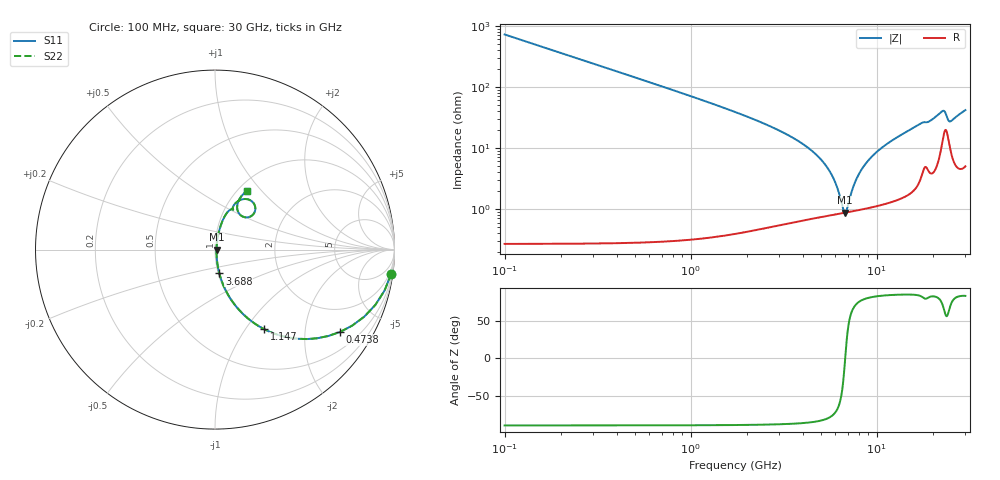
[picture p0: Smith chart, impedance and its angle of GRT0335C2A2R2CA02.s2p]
!Murata Part Number: GRT0335C2A2R2CA02
!These Parameters are Measured in Series Mode Connection
!Data Generated on Jun 19, 2026
!  o--ll--o
!Port1  Port2
!  o------o
!Operation Temp=25[degC], DC Bias Voltage=0[V]
!Freq. Start=100[MHz] Stop=30[GHz] 401[Steps]
# Hz S RI R 50
!Freq.(Hz) S11(Real) S11(Imag) S21(Real) S21(Imag) S12(Real) S12(Imag) S22(Real) S22(Imag)
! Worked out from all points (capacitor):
!   401 points, 100 MHz to 30 GHz, reference 50 ohm
!   read as one part in series: C = 2.2 pF near 249.5 MHz
!   lowest |Z| = 871 mohm at 6.753 GHz (marker M1)
!   series resonance near 6.776 GHz, so ESL is about 250 pH
!   S11 on the Smith chart (normalised r, x): 100 MHz: 1, -14; 473.8 MHz: 1.01, -3.04; 1.147 GHz: 1.01, -1.22; 3.688 GHz: 1.01, -0.27; 30 GHz: 1.10, +0.83
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1e8  0.9812 -0.1357  0.0188 0.1357  0.0188 0.1357  0.9812 -0.1357
3.2425e8  0.8317 -0.3735  0.1683 0.3735  0.1683 0.3735  0.8317 -0.3735
4.7375e8  0.6973 -0.4585  0.3027 0.4585  0.3027 0.4585  0.6973 -0.4585
7.7275e8  0.4602 -0.4968  0.5398 0.4968  0.5398 0.4968  0.4602 -0.4968
1.1465e9  0.2734 -0.443  0.7266 0.443  0.7266 0.443  0.2734 -0.443
2.0435e9  0.0961 -0.2882  0.9039 0.2882  0.9039 0.2882  0.0961 -0.2882
3.688e9  0.0241 -0.1326  0.9759 0.1326  0.9759 0.1326  0.0241 -0.1326
5.10825e9  0.0109 -0.0593  0.9891 0.0593  0.9891 0.0593  0.0109 -0.0593
5.9305e9  0.00879 -0.0277  0.9912 0.0277  0.9912 0.0277  0.00879 -0.0277
6.60325e9  0.00853 -0.00535  0.9915 0.00535  0.9915 0.00535  0.00853 -0.00535
6.75275e9  0.00861 -0.000705  0.9914 0.000705  0.9914 0.000705  0.00861 -0.000705
6.90225e9  0.00873 0.00384  0.9913 -0.00384  0.9913 -0.00384  0.00873 0.00384
7.575e9  0.00973 0.0232  0.9903 -0.0232  0.9903 -0.0232  0.00973 0.0232
8.09825e9  0.011 0.0372  0.989 -0.0372  0.989 -0.0372  0.011 0.0372
8.9205e9  0.0135 0.0577  0.9865 -0.0577  0.9865 -0.0577  0.0135 0.0577
1.01165e10  0.0184 0.0851  0.9816 -0.0851  0.9816 -0.0851  0.0184 0.0851
1.505e10  0.0525 0.1827  0.9475 -0.1827  0.9475 -0.1827  0.0525 0.1827
2.005825e10  0.1098 0.2538  0.8902 -0.2538  0.8902 -0.2538  0.1098 0.2538
2.26745e10  0.209 0.2657  0.791 -0.2657  0.791 -0.2657  0.209 0.2657
2.394525e10  0.1873 0.1807  0.8127 -0.1807  0.8127 -0.1807  0.1873 0.1807
2.50665e10  0.1294 0.2091  0.8706 -0.2091  0.8706 -0.2091  0.1294 0.2091
3e10  0.1761 0.3253  0.8239 -0.3253  0.8239 -0.3253  0.1761 0.3253
